{attribute 'pack_mode' := '1'}
TYPE ST_ReadListData_Array :
STRUCT
	stReadListReturnInfo	: ARRAY [1..2] OF ST_UAReadListReturnInfo;
	iArrayIntVar1 			: ARRAY[0..9] OF INT;
	iArrayIntVar2 			: ARRAY[0..11] OF INT;
END_STRUCT
END_TYPE
